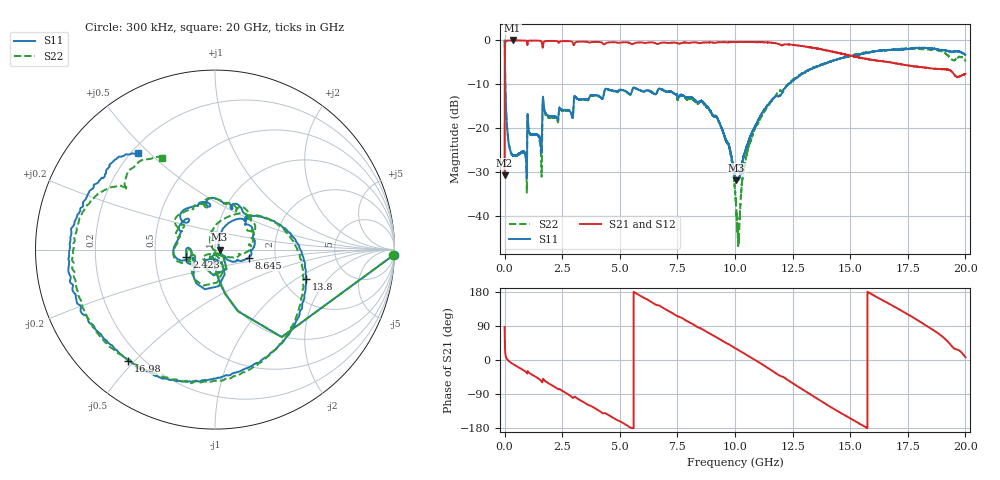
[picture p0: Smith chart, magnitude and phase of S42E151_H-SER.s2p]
! Created Wed Nov 25 22:00:22 2020
# khz S ma R 50
! 2 Port Network Data from SP1.SP block
! freq  magS11  angS11  magS21  angS21  magS12  angS12  magS22  angS22
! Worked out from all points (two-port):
!   20001 points, 300 kHz to 20 GHz, reference 50 ohm
!   highest |S21| = -0.01 dB at 348.3 MHz (marker M1); lowest = -30.7 dB at 300 kHz (marker M2)
!   |S21| within 3 dB of the highest: 10.36 MHz to 14.62 GHz (14.61 GHz wide, 200 % of centre); 14.62343 GHz to 14.62678 GHz (3.35 MHz wide, 0.0229 % of centre)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
!   lowest |S11| = -31.9 dB at 10.05 GHz (marker M3), VSWR 1.05, Z = 52.6 + j0.0541 ohm
!   |S11| at or under -10 dB: 31.02 MHz to 12.33 GHz (12.3 GHz wide, 199 % of centre); 12.33529 GHz to 12.33535 GHz (58.5 kHz wide, 0.000474 % of centre)
!   |S22| runs from -46.9 to -0.1 dB; largest |S21 - S12| = 0.018
!   S11 on the Smith chart (normalised r, x): 300 kHz: 8, -65; 2.423 GHz: 0.72, -0.06; 8.645 GHz: 1.46, -0.13; 13.8 GHz: 2.67, -1.20; 16.98 GHz: 0.15, -0.48; 20 GHz: 0.23, +0.46
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300  0.9961 -1.7  0.02901 87.4  0.0291 88.2  0.994 -1.8
104300  0.1036 -88.3  0.9937 2.1  0.9932 2.2  0.1042 -88.6
348300  0.04942 -100.3  0.9983 -10.0  0.997 -9.9  0.04903 -101.7
2423300  0.1652 -165.1  0.9751 -78.2  0.9753 -78.2  0.1623 -168.9
3334300  0.2125 158.8  0.9693 -108.1  0.9692 -108.0  0.2117 165.7
5191300  0.2673 100.1  0.9516 -168.1  0.9514 -168.1  0.2635 105.6
6667300  0.2748 67.9  0.9118 144.5  0.909 144.4  0.2753 59.5
8645300  0.1938 -13.3  0.9482 78.9  0.9472 78.9  0.1882 -1.9
9705300  0.06671 -34.4  0.9501 42.2  0.9511 42.2  0.06539 -32.4
1.00003e7  0.02821 -13.0  0.958 31.4  0.9581 31.4  0.01885 -57.6
1.00513e7  0.02547 1.2  0.9557 29.7  0.958 29.6  0.01222 -62.3
1.01663e7  0.02659 27.7  0.9578 25.7  0.9575 25.7  0.004983 -140.5
1.04313e7  0.05364 64.7  0.9574 16.1  0.9571 16.1  0.03959 126.3
1.09423e7  0.1131 69.7  0.954 -2.6  0.9535 -2.6  0.1083 97.7
1.23403e7  0.3182 34.8  0.898 -54.8  0.9008 -54.8  0.3234 34.3
1.33343e7  0.475 0.3  0.827 -93.1  0.8304 -92.9  0.4799 -6.3
1.38043e7  0.5323 -17.6  0.7864 -111.1  0.7928 -110.9  0.5374 -24.1
1.51573e7  0.6734 -69.8  0.6531 -159.2  0.6578 -159.9  0.6792 -69.1
1.66673e7  0.7758 -118.2  0.5674 149.2  0.5531 149.3  0.777 -122.1
1.69753e7  0.7871 -127.8  0.5463 138.6  0.5353 138.9  0.7885 -132.8
1.85263e7  0.8083 176.7  0.4776 82.0  0.4802 82.3  0.7853 175.7
2e7  0.6856 128.6  0.4156 7.3  0.4176 7.8  0.5868 119.8
